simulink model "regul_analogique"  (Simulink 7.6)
settings: Solver=ode23tb  StartTime=0.0  StopTime=20  FixedStep=Ts  RelTol=1e-3
InitFcn:
  | clc, close all,clear all
  | R=10; C=1e-6; L=1e-3;
  | Kp=0.1; Ki=1;
StopFcn:
  | close all
  | load Regul_PI.mat
  | plot(x(1,:),x(2,:), x(1,:),x(3,:), x(1,:),x(4,:))
  | grid
  | title('Signaux de la régulation PI')
  | axis([0 20 -2 12])
  | xlabel('temps')
libraries: powerlib x8

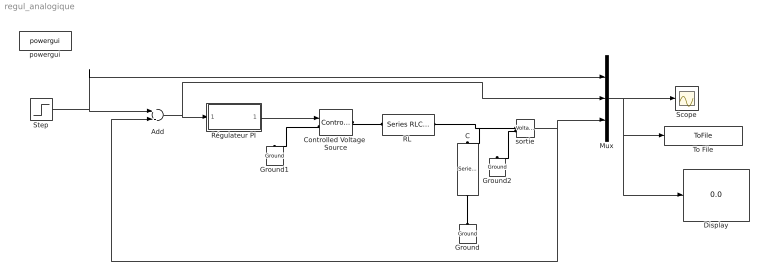
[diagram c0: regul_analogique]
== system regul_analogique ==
  Add : Sum  Inputs=+-
  C : powerlib/Elements/Series RLC Branch  DialogController=POWERSYS.PowerSysDialog  PhysicalDomain=powersysdomain  SubClassName=unknown  LeftPortType=p1  RightPortType=p1  LConnTagsString=__new0  RConnTagsString=__new0  BranchType=C  Resistance=10  Inductance=L  SetiL0=off  InitialCurrent=0  Capacitance=C  Setx0=off  InitialVoltage=0  Measurements=None
  Controlled Voltage  Source : powerlib/Electrical Sources/Controlled Voltage Source  DialogController=POWERSYS.PowerSysDialog  SystemSampleTime=-1  Initialize=on  Source_Type=AC  Amplitude=0  Phase=0  Frequency=0  Measurements=None
  Display : Display
  Ground : powerlib/Elements/Ground  DialogController=POWERSYS.PowerSysDialog  PhysicalDomain=powersysdomain  SubClassName=unknown  LeftPortType=p1  RightPortType=p1  LConnTagsString=a
  Ground1 : powerlib/Elements/Ground  DialogController=POWERSYS.PowerSysDialog  PhysicalDomain=powersysdomain  SubClassName=unknown  LeftPortType=p1  RightPortType=p1  LConnTagsString=a
  Ground2 : powerlib/Elements/Ground  DialogController=POWERSYS.PowerSysDialog  PhysicalDomain=powersysdomain  SubClassName=unknown  LeftPortType=p1  RightPortType=p1  LConnTagsString=a
  Mux : Mux  Inputs=3
  "RL " : powerlib/Elements/Series RLC Branch  DialogController=POWERSYS.PowerSysDialog  PhysicalDomain=powersysdomain  SubClassName=unknown  LeftPortType=p1  RightPortType=p1  LConnTagsString=__new0  RConnTagsString=__new0  BranchType=RL  Resistance=R  Inductance=1e-3  SetiL0=off  InitialCurrent=0  Capacitance=1e-6  Setx0=off  InitialVoltage=0  Measurements=None
  Régulateur PI : Subsystem
  Scope : Scope
  Step : Step  Time=5  After=10  SampleTime=0
  To File : ToFile  Filename=Regul_PI  MatrixName=x
  powergui : powerlib/powergui  SystemSampleTime=-1  SimulationMode=Continuous  SampleTime=0  frequency=60  SPID=off  DisableSnubberDevices=off  DisableRonSwitches=off  DisableVfSwitches=off  SwTol=0  Interpol=off  frequencyindice=0  echomessages=off  HookPort=off  DisplayEquations=off  FunctionMessages=off  EnableUseOfTLC=off  x0status=blocks  RestoreLinks=warning  ResistiveCurrentMeasurement=off  Frange=[0:2:500]  Ylog=off  Xlog=on  ShowGrid=off  save=off  variable=ZData  structure=ScopeData1  ZoomFFT=off  StartTime=0.0  cycles=1  DisplayStyle=1  fundamental=10  FreqAxis=off  MaxFrequency=100  frequencyindicesteady=60  RmsSteady=1  display=off  Ts=0  methode=off
  sortie : powerlib/Measurements/Voltage Measurement  DialogController=POWERSYS.PowerSysDialog  SystemSampleTime=-1  PhasorSimulation=off  OutputType=Complex  PSBequivalent=0
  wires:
  Step/1 -> Add/1, Mux/1
  sortie/1 -> Add/2, Mux/3
  Régulateur PI/1(cde) -> Controlled Voltage  Source/1
  Add/1 -> Régulateur PI/1(err), Mux/2
  Mux/1 -> Scope/1, To File/1, Display/1
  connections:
  Controlled Voltage  Source/RConn1 -- "RL "/LConn1
  Controlled Voltage  Source/LConn1 -- Ground1/LConn1
  sortie/LConn2 -- Ground2/LConn1
  C/RConn1 -- Ground/LConn1
  sortie/LConn1 -- "RL "/RConn1 -- C/LConn1

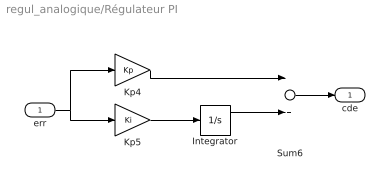
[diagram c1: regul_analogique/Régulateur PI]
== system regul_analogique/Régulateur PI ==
  err : Inport
  Integrator : Integrator
  Kp4 : Gain  Gain=Kp  SampleTime=0
  Kp5 : Gain  Gain=Ki  SampleTime=0
  Sum6 : Sum  SampleTime=0
  cde : Outport
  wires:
  Kp4/1 -> Sum6/1
  Kp5/1 -> Integrator/1
  Sum6/1 -> cde/1
  err/1 -> Kp4/1, Kp5/1
  Integrator/1 -> Sum6/2
